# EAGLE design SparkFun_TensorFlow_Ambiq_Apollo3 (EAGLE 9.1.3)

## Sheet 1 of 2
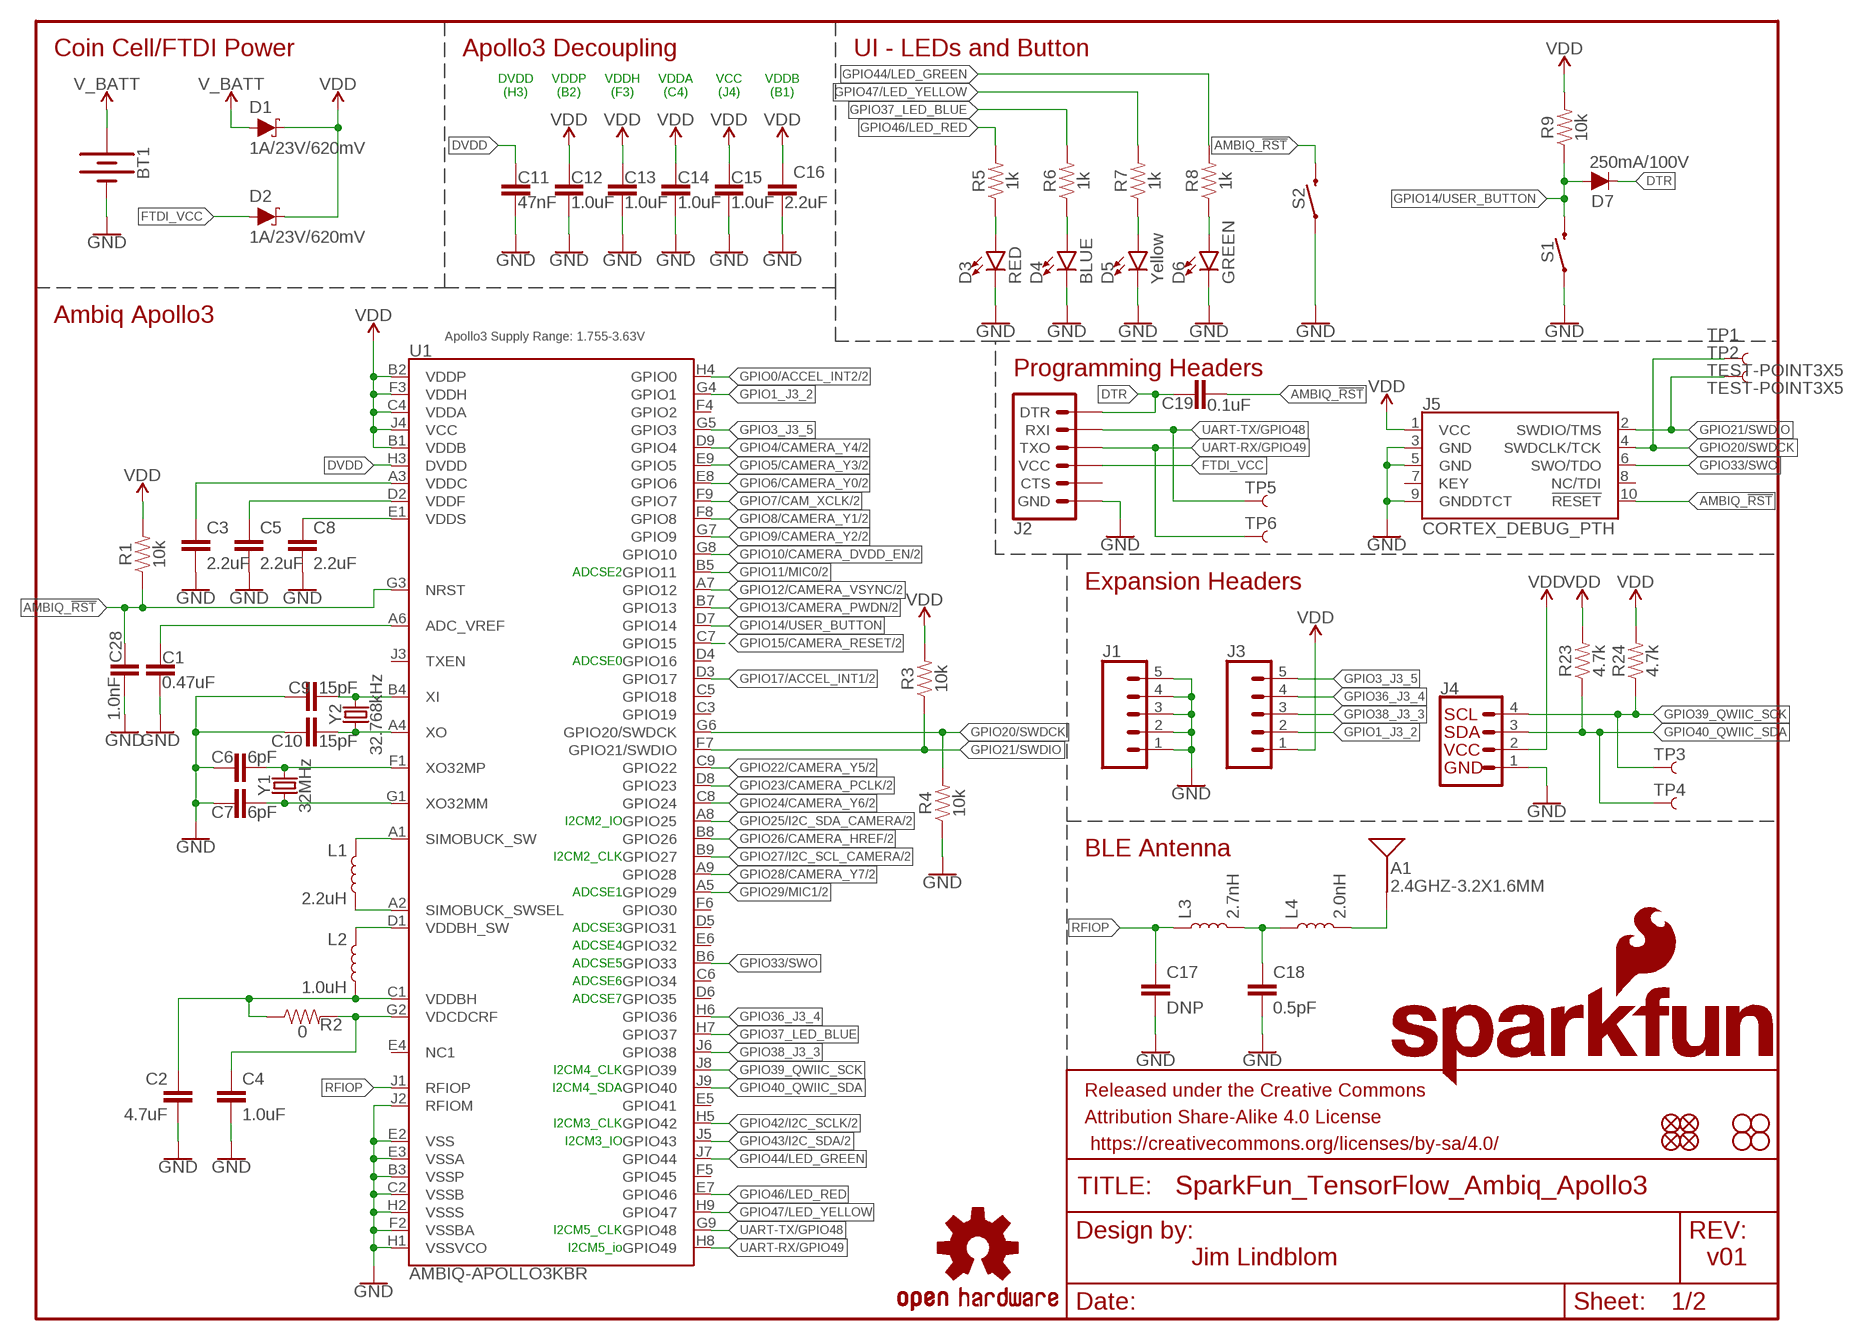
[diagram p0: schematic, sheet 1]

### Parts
A1  2.4GHZ-3.2X1.6MM  ANTENNA-2.4GHZ-3.2X1.6MM  [ANT-2.4GHZ-3.2X1.6X1.2MM]
BT1  BATTERY-20MM_SMD_4LEGS_OVERPASTE_INNER  [BATTCON_20MM_4LEGS_OVERPASTE_INNER]
C1  0.47uF  0.47UF-0402-TIGHT-6.3V-10%  [0402-TIGHT]
C2  4.7uF  4.7UF-0402-TIGHT-6.3V-(20%)  [0402-TIGHT]
C3  2.2uF  2.2UF-0402-TIGHT-25V-10%  [0402-TIGHT]
C4  1.0uF  1.0UF-0402-TIGHT-16V-10%  [0402-TIGHT]
C5  2.2uF  2.2UF-0402-TIGHT-25V-10%  [0402-TIGHT]
C6  6pF  6PF-0402-TIGHT-50V-0.5%  [0402-TIGHT]
C7  6pF  6PF-0402-TIGHT-50V-0.5%  [0402-TIGHT]
C8  2.2uF  2.2UF-0402-TIGHT-25V-10%  [0402-TIGHT]
C9  15pF  15PF-0402-TIGHT-50V-5%  [0402-TIGHT]
C10  15pF  15PF-0402-TIGHT-50V-5%  [0402-TIGHT]
C11  47nF  47NF-0402-TIGHT-25V-10%  [0402-TIGHT]
C12  1.0uF  1.0UF-0402-TIGHT-16V-10%  [0402-TIGHT]
C13  1.0uF  1.0UF-0402-TIGHT-16V-10%  [0402-TIGHT]
C14  1.0uF  1.0UF-0402-TIGHT-16V-10%  [0402-TIGHT]
C15  1.0uF  1.0UF-0402-TIGHT-16V-10%  [0402-TIGHT]
C16  2.2uF  2.2UF-0402-TIGHT-25V-10%  [0402-TIGHT]
C17  DNP  DNP-CAP-0402-TIGHT  [0402-TIGHT]
C18  0.5pF  0.5PF-0402-0.5PF-1%  [0402-TIGHT]
C19  0.1uF  0.1UF-0402-TIGHT-16V-10%  [0402-TIGHT]
C28  1.0nF  1.0NF/1000PF-0402-50V-10%  [0402-TIGHT]
D1  1A/23V/620mV  DIODE-SCHOTTKY-BAT20J  [SOD-323@1]
D2  1A/23V/620mV  DIODE-SCHOTTKY-BAT20J  [SOD-323@1]
D3  RED  LED-RED0603  [LED-0603]
D4  BLUE  LED-BLUE0603  [LED-0603]
D5  Yellow  LED-YELLOW0603  [LED-0603]
D6  GREEN  LED-GREEN0603  [LED-0603]
D7  250mA/100V  DIODE-BAS16J  [SOD-323]
FD1  FIDUCIAL1X2  [FIDUCIAL-1X2]
FD2  FIDUCIAL1X2  [FIDUCIAL-1X2]
FD3  FIDUCIAL1X2  [FIDUCIAL-1X2]
FD4  FIDUCIAL1X2  [FIDUCIAL-1X2]
FRAME1  FRAME-LETTER  [CREATIVE_COMMONS]
H1  STAND-OFF  [STAND-OFF]
H2  STAND-OFF  [STAND-OFF]
H3  STAND-OFF  [STAND-OFF]
H4  STAND-OFF  [STAND-OFF]
J1  CONN_05NO_SILK  [1X05_NO_SILK]
J2  6_PIN_SERIAL_TARGETSMD  [1X06-SMD_RA_MALE]
J3  CONN_05NO_SILK  [1X05_NO_SILK]
J4  QWIIC_CONNECTORJS-1MM  [1X04_1MM_RA]
J5  CORTEX_DEBUG_PTH  [2X5-PTH-1.27MM]
L1  2.2uH  INDUCTOR-0805-2.2UH  [0805-WIDE]
L2  1.0uH  INDUCTOR-0805-1.0UH  [0805-WIDE]
L3  2.7nH  INDUCTOR-0402-2.7NH  [0402-TIGHT]
L4  2.0nH  INDUCTOR-0402-2.0NH  [0402-TIGHT]
LOGO1  SFE_LOGO_NAME_FLAME.1_INCH  [SFE_LOGO_NAME_FLAME_.1]
LOGO2  OSHW-LOGOS  [OSHW-LOGO-S]
R1  10k  10KOHM-0402-TIGHT-1/10W-1%  [0402-TIGHT]
R2  0  0OHM-0402-TIGHT-1/10W-5%  [0402-TIGHT]
R3  10k  10KOHM-0402-TIGHT-1/10W-1%  [0402-TIGHT]
R4  10k  10KOHM-0402-TIGHT-1/10W-1%  [0402-TIGHT]
R5  1k  1KOHM-0603-1/10W-1%  [0603]
R6  1k  1KOHM-0603-1/10W-1%  [0603]
R7  1k  1KOHM-0603-1/10W-1%  [0603]
R8  1k  1KOHM-0603-1/10W-1%  [0603]
R9  10k  10KOHM-0402-TIGHT-1/10W-1%  [0402-TIGHT]
R23  4.7k  4.7KOHM-0603-1/10W-1%  [0603]
R24  4.7k  4.7KOHM-0603-1/10W-1%  [0603]
S1  MOMENTARY-SWITCH-SPST-SMD-5.2-TALL-REDUNDANT  [TACTILE_SWITCH_SMD_5.2MM]
S2  MOMENTARY-SWITCH-SPST-SMD-5.2-TALL-REDUNDANT  [TACTILE_SWITCH_SMD_5.2MM]
TP1  TEST-POINT3X5  [PAD.03X.05]
TP2  TEST-POINT3X5  [PAD.03X.05]
TP3  TEST-POINT3X5  [PAD.03X.05]
TP4  TEST-POINT3X5  [PAD.03X.05]
TP5  TEST-POINT3X5  [PAD.03X.05]
TP6  TEST-POINT3X5  [PAD.03X.05]
U1  AMBIQ-APOLLO3KBR  [BGA-81-5X5MM]
Y1  32MHz  CRYSTAL-32MHZ-SMD-2.0X1.6MM  [CRYSTAL-SMD-2.0X1.6MM]
Y2  32.768kHz  CRYSTAL-32.768KHZSMD-3.2X1.5  [CRYSTAL-SMD-3.2X1.5MM]

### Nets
ADC_VREF: C1.1 U1.A6(ADC_VREF)
AMBIQ_!RST: C19.2 C28.1 J5.10(!RESET) R1.1 S2.3 S2.4 U1.G3(NRST)
DTR: C19.1 D7.C J2.1(DTR)
DVDD: C11.1 U1.H3(DVDD)
FTDI_VCC: D2.A J2.4(VCC)
GND: BT1.2(-) C1.2 C2.2 C3.2 C4.2 C5.2 C6.1 C7.1 C8.2 C9.1 C10.1 C11.2 C12.2 C13.2 C14.2 C15.2 C16.2 C17.2 C18.2 C28.2 D3.C D4.C D5.C D6.C J1.1 J1.2 J1.3 J1.4 J1.5 J2.6(GND) J4.1 J5.3(GND) J5.5(GND) J5.9(GNDDTCT) R4.1 S1.1 S1.2 S2.1 S2.2 U1.B3(VSSP) U1.C2(VSSB) U1.E2(VSS) U1.E3(VSSA) U1.F2(VSSBA) U1.H1(VSSVCO) U1.H2(VSSS) U1.J2(RFIOM) ; also sheet 2
GPIO0/ACCEL_INT2: U1.H4(GPIO0) ; also sheet 2
GPIO1_J3_2: J3.2 U1.G4(GPIO1)
GPIO3_J3_5: J3.5 U1.G5(GPIO3)
GPIO4/CAMERA_Y4: U1.D9(GPIO4) ; also sheet 2
GPIO5/CAMERA_Y3: U1.E9(GPIO5) ; also sheet 2
GPIO6/CAMERA_Y0: U1.E8(GPIO6) ; also sheet 2
GPIO7/CAM_XCLK: U1.F9(GPIO7) ; also sheet 2
GPIO8/CAMERA_Y1: U1.F8(GPIO8) ; also sheet 2
GPIO9/CAMERA_Y2: U1.G7(GPIO9) ; also sheet 2
GPIO10/CAMERA_DVDD_EN: U1.G8(GPIO10) ; also sheet 2
GPIO11/MIC0: U1.B5(GPIO11) ; also sheet 2
GPIO12/CAMERA_VSYNC: U1.A7(GPIO12) ; also sheet 2
GPIO13/CAMERA_PWDN: U1.B7(GPIO13) ; also sheet 2
GPIO14/USER_BUTTON: D7.A R9.1 S1.3 S1.4 U1.D7(GPIO14)
GPIO15/CAMERA_RESET: U1.C7(GPIO15) ; also sheet 2
GPIO17/ACCEL_INT1: U1.D3(GPIO17) ; also sheet 2
GPIO20/SWDCK: J5.4(SWDCLK/TCK) R4.2 TP1.P$1 U1.G6(GPIO20/SWDCK)
GPIO21/SWDIO: J5.2(SWDIO/TMS) R3.1 TP2.P$1 U1.F7(GPIO21/SWDIO)
GPIO22/CAMERA_Y5: U1.C9(GPIO22) ; also sheet 2
GPIO23/CAMERA_PCLK: U1.D8(GPIO23) ; also sheet 2
GPIO24/CAMERA_Y6: U1.C8(GPIO24) ; also sheet 2
GPIO25/I2C_SDA_CAMERA: U1.A8(GPIO25) ; also sheet 2
GPIO26/CAMERA_HREF: U1.B8(GPIO26) ; also sheet 2
GPIO27/I2C_SCL_CAMERA: U1.B9(GPIO27) ; also sheet 2
GPIO28/CAMERA_Y7: U1.A9(GPIO28) ; also sheet 2
GPIO29/MIC1: U1.A5(GPIO29) ; also sheet 2
GPIO33/SWO: J5.6(SWO/TDO) U1.B6(GPIO33)
GPIO36_J3_4: J3.4 U1.H6(GPIO36)
GPIO37_LED_BLUE: R6.2 U1.H7(GPIO37)
GPIO38_J3_3: J3.3 U1.J6(GPIO38)
GPIO39_QWIIC_SCK: J4.4 R24.1 TP3.P$1 U1.J8(GPIO39)
GPIO40_QWIIC_SDA: J4.3 R23.1 TP4.P$1 U1.J9(GPIO40)
GPIO42/I2C_SCLK: U1.H5(GPIO42) ; also sheet 2
GPIO43/I2C_SDA: U1.J5(GPIO43) ; also sheet 2
GPIO44/LED_GREEN: R8.2 U1.J7(GPIO44)
GPIO46/LED_RED: R5.2 U1.E7(GPIO46)
GPIO47/LED_YELLOW: R7.2 U1.H9(GPIO47)
N$1: A1.FEED(SIGNAL) L4.2
N$2: C7.2 U1.G1(XO32MM) Y1.1
N$3: C6.2 U1.F1(XO32MP) Y1.3
N$5: D4.A R6.1
N$6: D3.A R5.1
N$7: D5.A R7.1
N$8: D6.A R8.1
N$16: C18.1 L3.2 L4.1
RFIOP: C17.1 L3.1 U1.J1(RFIOP)
SIMBUCK_SWSEL: L1.2 U1.A2(SIMOBUCK_SWSEL)
SIMOBUCK_SW: L1.1 U1.A1(SIMOBUCK_SW)
UART-RX/GPIO49: J2.3(TXO) TP6.P$1 U1.H8(GPIO49)
UART-TX/GPIO48: J2.2(RXI) TP5.P$1 U1.G9(GPIO48)
V_BATT: BT1.1(+) D1.A
VDCDCRF: C4.1 R2.2 U1.G2(VDCDCRF)
VDD: C12.1 C13.1 C14.1 C15.1 C16.1 D1.C D2.C J3.1 J4.2 J5.1(VCC) R1.2 R3.2 R9.2 R23.2 R24.2 U1.B1(VDDB) U1.B2(VDDP) U1.C4(VDDA) U1.F3(VDDH) U1.J4(VCC) ; also sheet 2
VDDBH: C2.1 L2.2 R2.1 U1.C1(VDDBH)
VDDBH_SW: L2.1 U1.D1(VDDBH_SW)
VDDC: C3.1 U1.A3(VDDC)
VDDF: C5.1 U1.D2(VDDF)
VDDS: C8.1 U1.E1(VDDS)
X0: C10.2 U1.A4(XO) Y2.P$1
XI: C9.2 U1.B4(XI) Y2.P$2
Unconnected: J2.5(CTS) J5.7(KEY) J5.8(NC/TDI) U1.C3(GPIO19) U1.C5(GPIO18) U1.C6(GPIO34) U1.D4(GPIO16) U1.D5(GPIO31) U1.D6(GPIO35) U1.E4(NC1) U1.E5(GPIO41) U1.E6(GPIO32) U1.F4(GPIO2) U1.F5(GPIO45) U1.F6(GPIO30) U1.J3(TXEN)

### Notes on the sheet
- Coin Cell/FTDI Power | Apollo3 Decoupling | UI - LEDs and Button
- DVDD
  (H3)
- VDDP
  (B2)
- VDDH
  (F3)
- VDDA
  (C4)
- VCC
  (J4)
- VDDB
  (B1)
- Ambiq Apollo3
- Apollo3 Supply Range: 1.755-3.63V
- Programming Headers
- ADCSE2 | Expansion Headers
- ADCSE0
- I2CM2_IO
- BLE Antenna
- I2CM2_CLK
- ADCSE1
- ADCSE3
- ADCSE4
- ADCSE5
- ADCSE6
- ADCSE7
- I2CM4_CLK
- I2CM4_SDA
- I2CM3_CLK
- I2CM3_IO
- I2CM5_CLK
- I2CM5_io | Jim Lindblom | v01

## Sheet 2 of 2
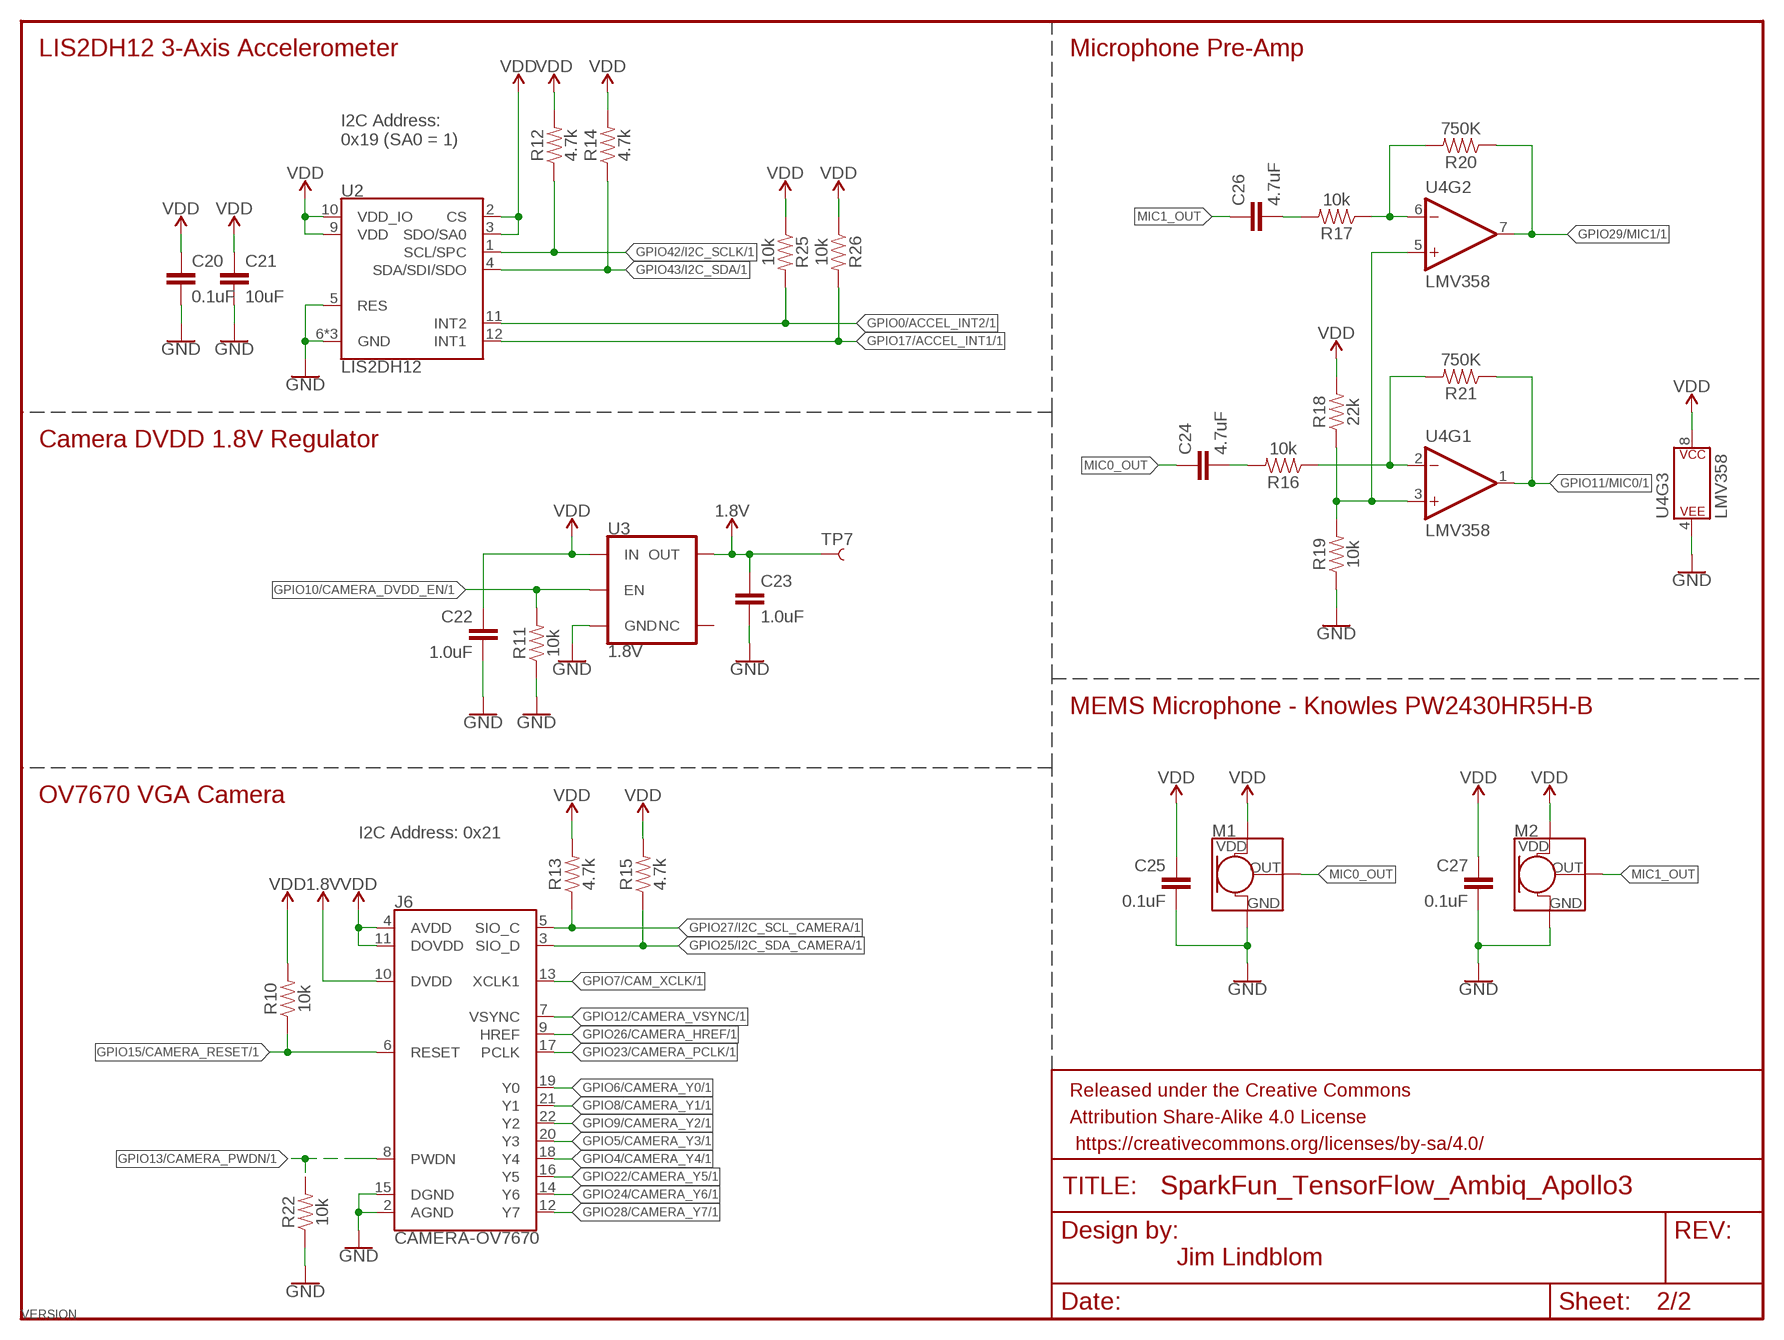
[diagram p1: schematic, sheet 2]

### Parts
C20  0.1uF  0.1UF-0402-TIGHT-16V-10%  [0402-TIGHT]
C21  10uF  10UF-0603-6.3V-20%  [0603]
C22  1.0uF  1.0UF-0402-TIGHT-16V-10%  [0402-TIGHT]
C23  1.0uF  1.0UF-0402-TIGHT-16V-10%  [0402-TIGHT]
C24  4.7uF  4.7UF-0603-6.3V-(10%)  [0603]
C25  0.1uF  0.1UF-0402-TIGHT-16V-10%  [0402-TIGHT]
C26  4.7uF  4.7UF-0603-6.3V-(10%)  [0603]
C27  0.1uF  0.1UF-0402-TIGHT-16V-10%  [0402-TIGHT]
FRAME2  FRAME-LETTERNO_PACKAGE  [DUMMY]
J6  CAMERA-OV7670  [FPC-24-AMPHENOL-SFV24R-1STE1HLF]
M1  MEMS_MIC  MEMS_MICROPHONESPW2430HR5H-B  [SPW2430HR5H-B]
M2  MEMS_MIC  MEMS_MICROPHONESPW2430HR5H-B  [SPW2430HR5H-B]
R10  10k  10KOHM-0402-TIGHT-1/10W-1%  [0402-TIGHT]
R11  10k  10KOHM-0402-TIGHT-1/10W-1%  [0402-TIGHT]
R12  4.7k  4.7KOHM-0603-1/10W-1%  [0603]
R13  4.7k  4.7KOHM-0603-1/10W-1%  [0603]
R14  4.7k  4.7KOHM-0603-1/10W-1%  [0603]
R15  4.7k  4.7KOHM-0603-1/10W-1%  [0603]
R16  10k  10KOHM-0603-1/10W-1%  [0603]
R17  10k  10KOHM-0603-1/10W-1%  [0603]
R18  22k  22KOHM-0402-1/16W-1%  [0402-TIGHT]
R19  10k  10KOHM-0402-TIGHT-1/10W-1%  [0402-TIGHT]
R20  750K  750KOHM-0603-1/10W-1%  [0603]
R21  750K  750KOHM-0603-1/10W-1%  [0603]
R22  10k  10KOHM-0402-TIGHT-1/10W-1%  [0402-TIGHT]
R25  10k  10KOHM-0402-TIGHT-1/10W-1%  [0402-TIGHT]
R26  10k  10KOHM-0402-TIGHT-1/10W-1%  [0402-TIGHT]
TP7  TEST-POINT3X5  [PAD.03X.05]
U2  LIS2DH12  [LGA-12-LISDH12]
U3  1.8V  V_REG_AP2127K-2.8  [SOT23-5]
U4  LMV358  LMV358SOIC  [SO08]

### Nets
1.8V: C23.1 J6.10(DVDD) TP7.P$1 U3.5(OUT)
GND: C20.2 C21.2 C22.2 C23.2 C25.2 C27.2 J6.2(AGND) J6.15(DGND) M1.2(GND) M1.3(GND) M2.2(GND) M2.3(GND) R11.1 R19.1 R22.1 U2.5(RES) U2.6(GND) U2.7(GND) U2.8(GND) U3.2(GND) U4.4(P$V-) ; also sheet 1
GPIO0/ACCEL_INT2: R25.2 U2.11(INT2) ; also sheet 1
GPIO4/CAMERA_Y4: J6.18(Y4) ; also sheet 1
GPIO5/CAMERA_Y3: J6.20(Y3) ; also sheet 1
GPIO6/CAMERA_Y0: J6.19(Y0) ; also sheet 1
GPIO7/CAM_XCLK: J6.13(XCLK1) ; also sheet 1
GPIO8/CAMERA_Y1: J6.21(Y1) ; also sheet 1
GPIO9/CAMERA_Y2: J6.22(Y2) ; also sheet 1
GPIO10/CAMERA_DVDD_EN: R11.2 U3.3(EN) ; also sheet 1
GPIO11/MIC0: R21.1 U4.1(OUT) ; also sheet 1
GPIO12/CAMERA_VSYNC: J6.7(VSYNC) ; also sheet 1
GPIO13/CAMERA_PWDN: J6.8(PWDN) R22.2 ; also sheet 1
GPIO15/CAMERA_RESET: J6.6(RESET) R10.1 ; also sheet 1
GPIO17/ACCEL_INT1: R26.2 U2.12(INT1) ; also sheet 1
GPIO22/CAMERA_Y5: J6.16(Y5) ; also sheet 1
GPIO23/CAMERA_PCLK: J6.17(PCLK) ; also sheet 1
GPIO24/CAMERA_Y6: J6.14(Y6) ; also sheet 1
GPIO25/I2C_SDA_CAMERA: J6.3(SIO_D) R15.1 ; also sheet 1
GPIO26/CAMERA_HREF: J6.9(HREF) ; also sheet 1
GPIO27/I2C_SCL_CAMERA: J6.5(SIO_C) R13.1 ; also sheet 1
GPIO28/CAMERA_Y7: J6.12(Y7) ; also sheet 1
GPIO29/MIC1: R20.1 U4.7(OUT) ; also sheet 1
GPIO42/I2C_SCLK: R12.1 U2.1(SCL/SPC) ; also sheet 1
GPIO43/I2C_SDA: R14.1 U2.4(SDA/SDI/SDO) ; also sheet 1
MIC0_OUT: C24.1 M1.1(OUT)
MIC1_OUT: C26.1 M2.1(OUT)
N$9: R18.1 R19.2 U4.3(+IN) U4.5(+IN)
N$10: C24.2 R16.2
N$11: R17.1 R20.2 U4.6(-IN)
N$12: R16.1 R21.2 U4.2(-IN)
N$14: C26.2 R17.2
VDD: C20.1 C21.1 C22.1 C25.1 C27.1 J6.4(AVDD) J6.11(DOVDD) M1.4(VDD) M2.4(VDD) R10.2 R12.2 R13.2 R14.2 R15.2 R18.2 R25.1 R26.1 U2.2(CS) U2.3(SDO/SA0) U2.9(VDD) U2.10(VDD_IO) U3.1(IN) U4.8(P$V+) ; also sheet 1
Unconnected: J6.MNT1@0(MNT1) J6.MNT1@1(MNT1) J6.MNT2@0(MNT2) J6.MNT2@1(MNT2) U3.4(NC)

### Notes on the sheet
- LIS2DH12 3-Axis Accelerometer | Microphone Pre-Amp
- I2C Address:
  0x19 (SA0 = 1)
- Camera DVDD 1.8V Regulator
- MEMS Microphone - Knowles PW2430HR5H-B
- OV7670 VGA Camera
- I2C Address: 0x21
- Jim Lindblom

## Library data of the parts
A1 = ambiq:ANTENNA: Single-ended Antennae; DIGIKEY: 535-14095-2-ND; PROD_ID: ANT-14235
BT1 = SparkFun-Batteries:BATTERY: Battery - Single Cell
C1 = ambiq:0.47UF: 0.47uF ceramic capacitor; DIGIKEY: 1276-1479-2-ND
C2 = ambiq:4.7UF: 4.7µF ceramic capacitors; DIGIKEY: 1276-1056-1-ND
C3 C5 C8 C16 = ambiq:2.2UF: 2.2µF ceramic capacitors; DIGIKEY: 1276-1462-2-ND
C4 C12-C15 C22 C23 = ambiq:1.0UF: 1µF ceramic capacitors; PROD_ID: CAP-12417
C6 C7 = ambiq:6PF: 6pF ceramic capacitors; PROD_ID: CAP-13455
C9 C10 = ambiq:15PF: 15pF ceramic capacitors; PROD_ID: CAP-13063
C11 = ambiq:47NF: 47nF ceramic capacitors; DIGIKEY: 311-1717-2-ND
C17 = ambiq:DNP-CAP: 0.18µF ceramic capacitor
C18 = ambiq:0.5PF: 0.5pF ceramic capacitor; DIGIKEY: 399-16299-1-ND
C19 C20 C25 C27 = ambiq:0.1UF: 0.1µF ceramic capacitors; PROD_ID: CAP-12416
C21 = SparkFun-Capacitors:10UF: 10.0µF ceramic capacitors; PROD_ID: CAP-11015
C24 C26 = SparkFun-Capacitors:4.7UF: 4.7µF ceramic capacitors; PROD_ID: CAP-08280
C28 = ambiq:1.0NF/1000PF: 1nF/1,000pF ceramic capacitors; DIGIKEY: 311-1036-2-ND
D1 D2 = SparkFun-DiscreteSemi:DIODE-SCHOTTKY: Schottky diode; PROD_ID: DIO-11623
D3 = SparkFun-LED:LED-RED: Red SMD LED; PROD_ID: DIO-00819
D4 = SparkFun-LED:LED-BLUE: Blue SMD LED; PROD_ID: DIO-08575
D5 = SparkFun-LED:LED-YELLOW: Yellow SMD LED; PROD_ID: DIO-09003
D6 = SparkFun-LED:LED-GREEN: Green SMD LED; PROD_ID: DIO-00821
D7 = SparkFun-DiscreteSemi:DIODE: Diode; PROD_ID: DIO-09646
FD1-FD4 = SparkFun-Aesthetics:FIDUCIAL: Fiducial Alignment Points
FRAME1 = SparkFun-Aesthetics:FRAME-LETTER: Schematic Frame - Letter
FRAME2 = SparkFun-Aesthetics:FRAME-LETTER: Schematic Frame - Letter; DESIGNER: Nobody; VERSION: x01
H1-H4 = SparkFun-Hardware:STAND-OFF: Stand Off
J1 J3 = SparkFun-Connectors:CONN_05: Multi connection point. Often used as Generic Header-pin footprint for 0.1 inch spaced/style header connections On any of the 0.1 inch spaced packages, you can populate with these: Break Away Headers - Straight (PRT-00116) Break Away Male Headers - Right Angle (PRT-00553) Female Headers (PRT-00115)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
J2 = SparkFun-Connectors:6_PIN_SERIAL_TARGET: 6-pin header connection for use with the "FTDI BASIC" pinout - TARGET SIDE. Also known as "Arduino Serial Program Header". It is used to mate with our FTDI Basic serial programmers using the Arduino IDE. Note, this device has "TARGET" in the name. It is intended to be used on a design that contains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; PROD_ID: CONN-08971
J4 = SparkFun-Connectors:QWIIC_CONNECTOR: SparkFun I2C Standard Qwiic Connector An SMD 1mm pitch JST connector makes it easy and quick (get it? Qwiic?) to connect I2C devices to each other. The Qwiic system enables fast and solderless connection between popular platforms and various sensors and actuators. We carry 200mm, 100mm, 50mm, and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; PROD_ID: CONN-13694
J5 = SparkFun-Connectors:CORTEX_DEBUG: Cortex Debug Connector - 10 pin Supports JTAG debug, Serial Wire debug, and Serial Wire Viewer. PTH and SMD connector options available. General Connector Information Products: PTH Connector -via Digi-Key SparkFun PSoc SparkFun T
J6 = ambiq:CAMERA-OV7670; DIGIKEY: 609-4320-2-ND
L1 = ambiq:INDUCTOR: Inductors; DIGIKEY: 490-17728-2-ND
L2 = ambiq:INDUCTOR: Inductors; DIGIKEY: 587-2903-2-ND
L3 = ambiq:INDUCTOR: Inductors; DIGIKEY: 445-172420-1-ND
L4 = ambiq:INDUCTOR: Inductors; DIGIKEY: 490-6752-1-ND
LOGO1 = SparkFun-Aesthetics:SFE_LOGO_NAME_FLAME: SparkFun Font Logo w/ Flame
LOGO2 = SparkFun-Aesthetics:OSHW-LOGO: Open-Source Hardware (OSHW) Logo
M1 M2 = ambiq:MEMS_MICROPHONE; DIGIKEY: 423-1394-2-ND
R1 R3 R4 R9-R11 R19 R22 R25 R26 = ambiq:10KOHM: 10kΩ resistor; DIGIKEY: 311-10.0KLRTR-ND
R2 = ambiq:0OHM: 0Ω resistor; DIGIKEY: 311-0.0JRTR-ND
R5-R8 = SparkFun-Resistors:1KOHM: 1kΩ resistor; PROD_ID: RES-07856
R12-R15 R23 R24 = SparkFun-Resistors:4.7KOHM: 4.7kΩ resistor; PROD_ID: RES-07857
R16 R17 = SparkFun-Resistors:10KOHM: 10kΩ resistor; PROD_ID: RES-00824
R18 = ambiq:22KOHM: 22kΩ resistor; DIGIKEY: 311-22.0KLRTR-ND
R20 R21 = SparkFun-Resistors:750KOHM: 750Ω resistor; PROD_ID: RES-13768
S1 S2 = SparkFun-Switches:MOMENTARY-SWITCH-SPST: Momentary Switch (Pushbutton) - SPST; PROD_ID: SWCH-14139
TP1-TP7 = SparkFun-Connectors:TEST-POINT: SparkFun Test Points
U1 = ambiq:AMBIQ-APOLLO3
U2 = ambiq:LIS2DH12; DIGIKEY: 497-14851-2-ND
U3 = ambiq:V_REG_AP2127: Diodes Inc AP2127 -- 300mA LDO Regulator Datasheet; DIGIKEY: AP2127K-1.8TRG1DITR-ND
U4 = SparkFun-IC-Amplifiers:LMV358: IC LMV358 DUAL OP AMP Jellybean rail-to-rail output op-amp SparkFun Products SparkFun PicoBoard (WIG-11888) SparkFun Vernier Interface Shield (DEV-12858) SparkFun Blynk Board - ESP8266 (WRL-13794) SparkFun Digital Sandbox (DEV-12651 RoHS); PROD_ID: IC-09657
Y1 = SparkFun-Clocks:CRYSTAL-32MHZ: 32MHz Crystal; PROD_ID: XTAL-13459
Y2 = SparkFun-Clocks:CRYSTAL-32.768KHZ: 32.768kHz Crystal; PROD_ID: XTAL-13062

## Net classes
0 default: width 0 mm, drill 0 mm
2 usb: width 0.254 mm, drill 0.305 mm, clearance 0.254 mm

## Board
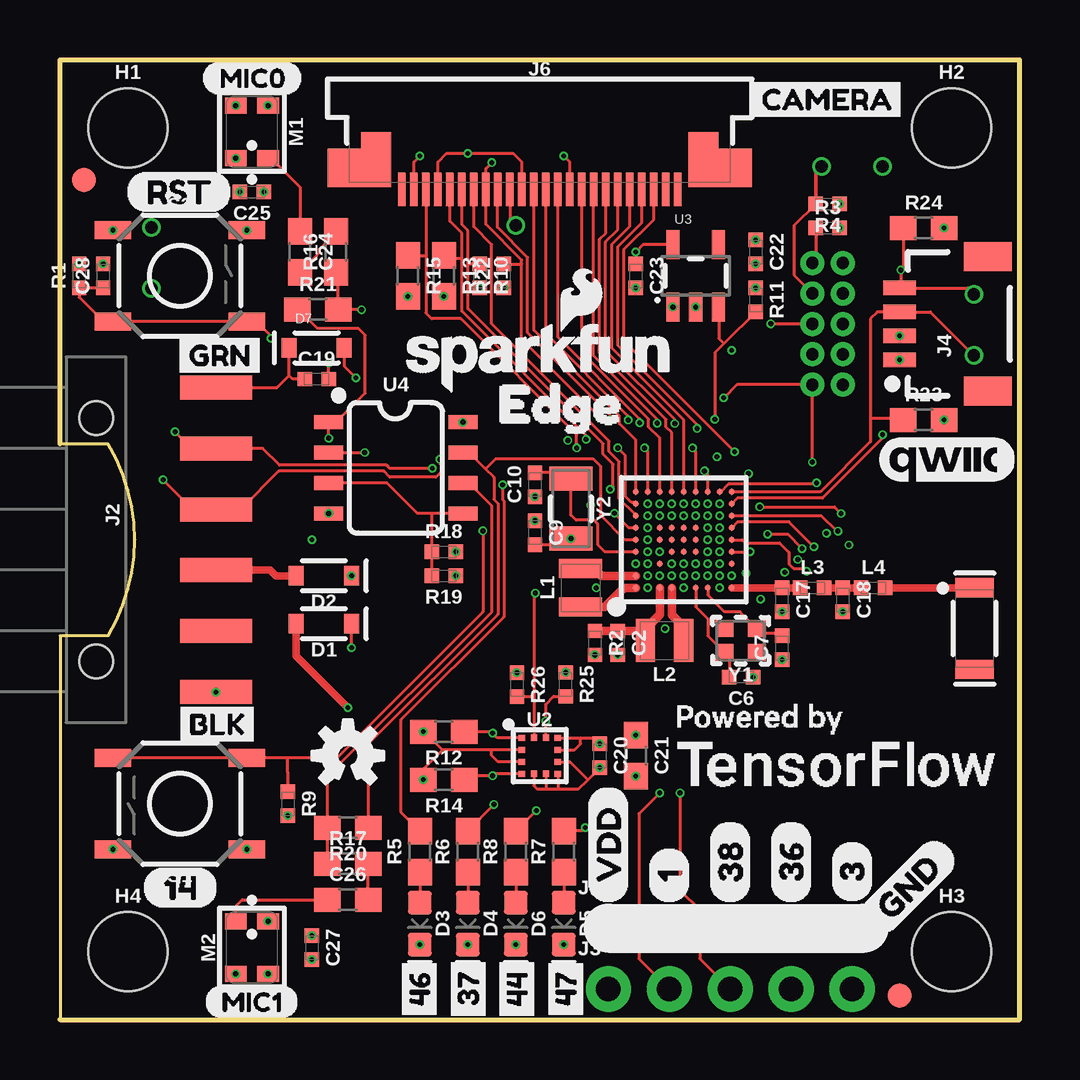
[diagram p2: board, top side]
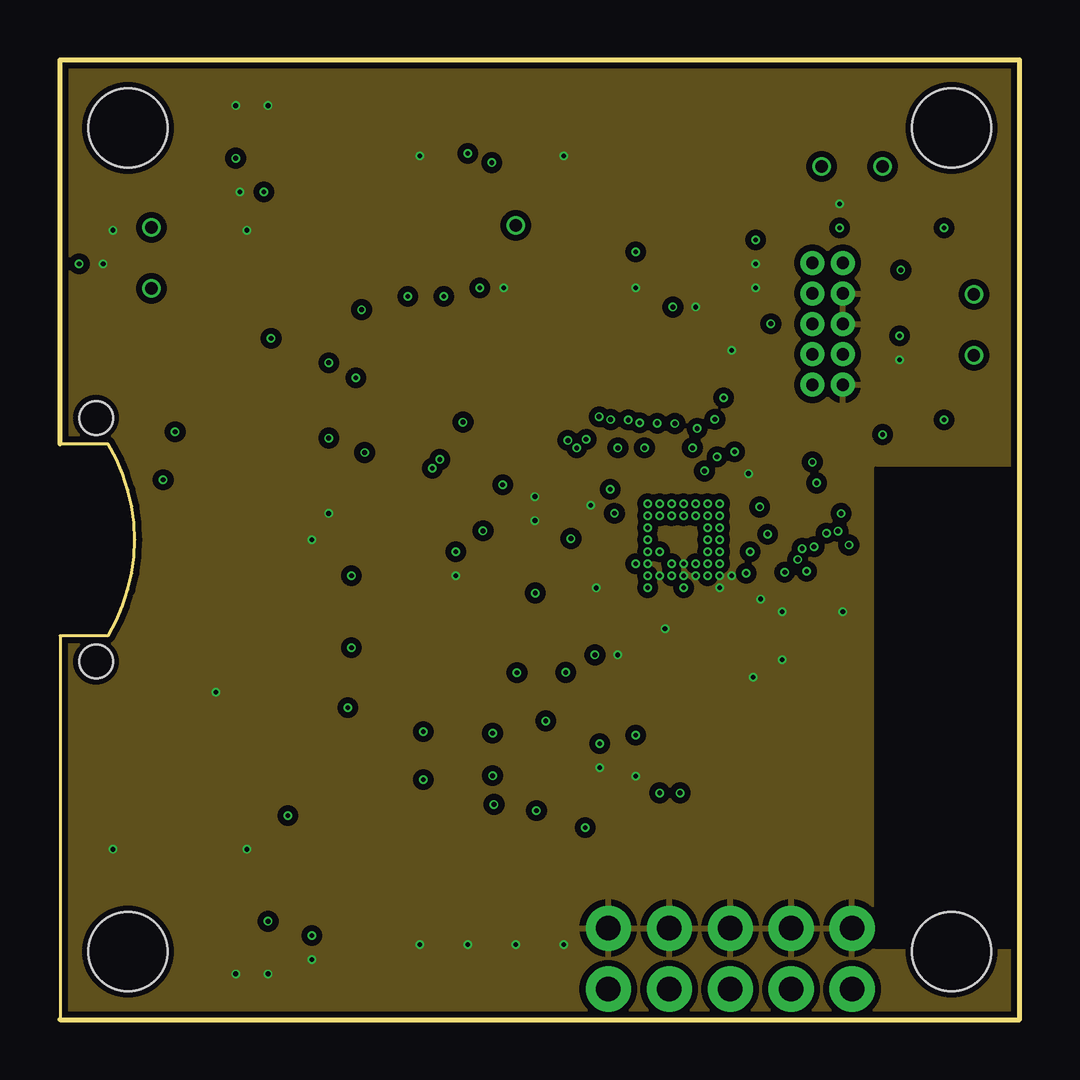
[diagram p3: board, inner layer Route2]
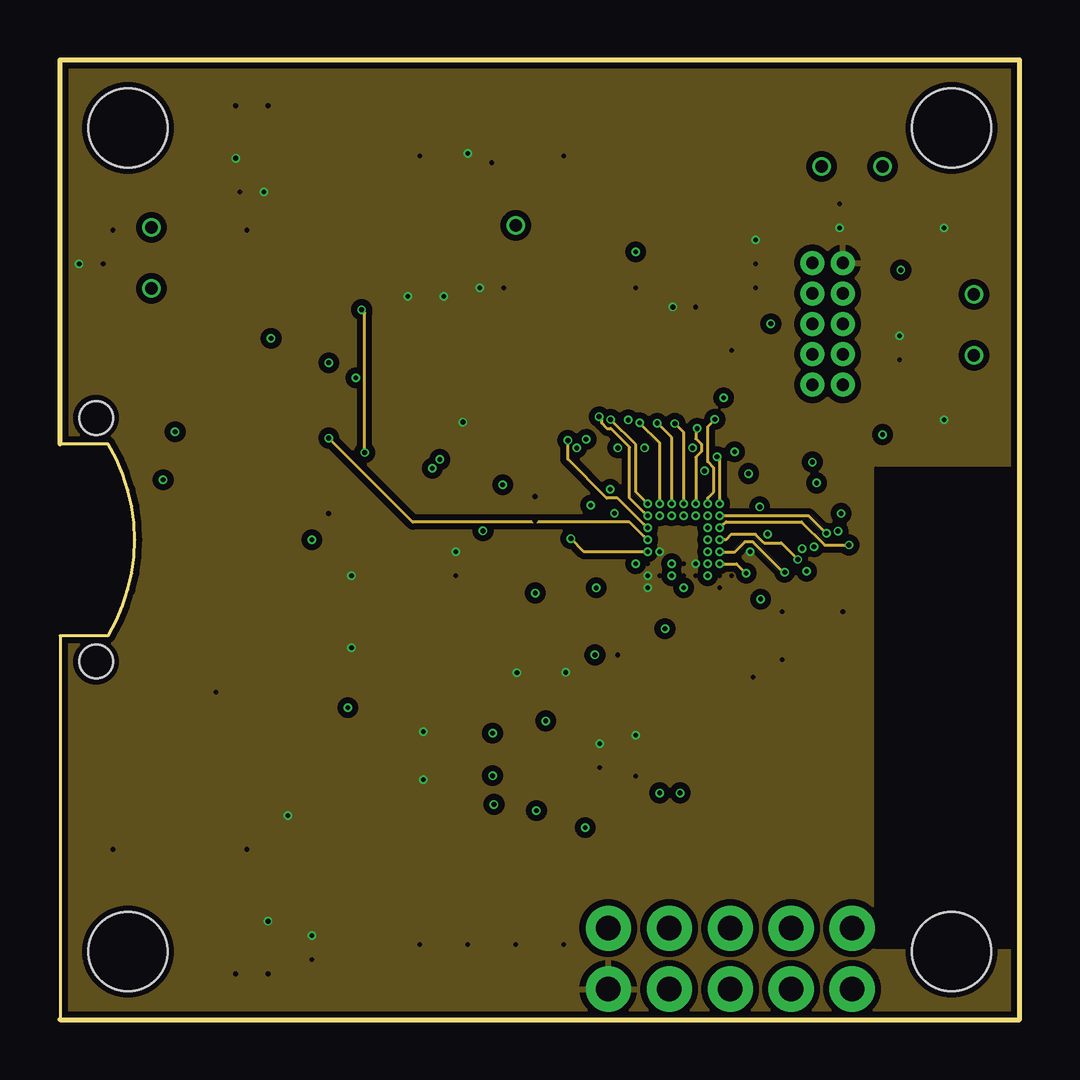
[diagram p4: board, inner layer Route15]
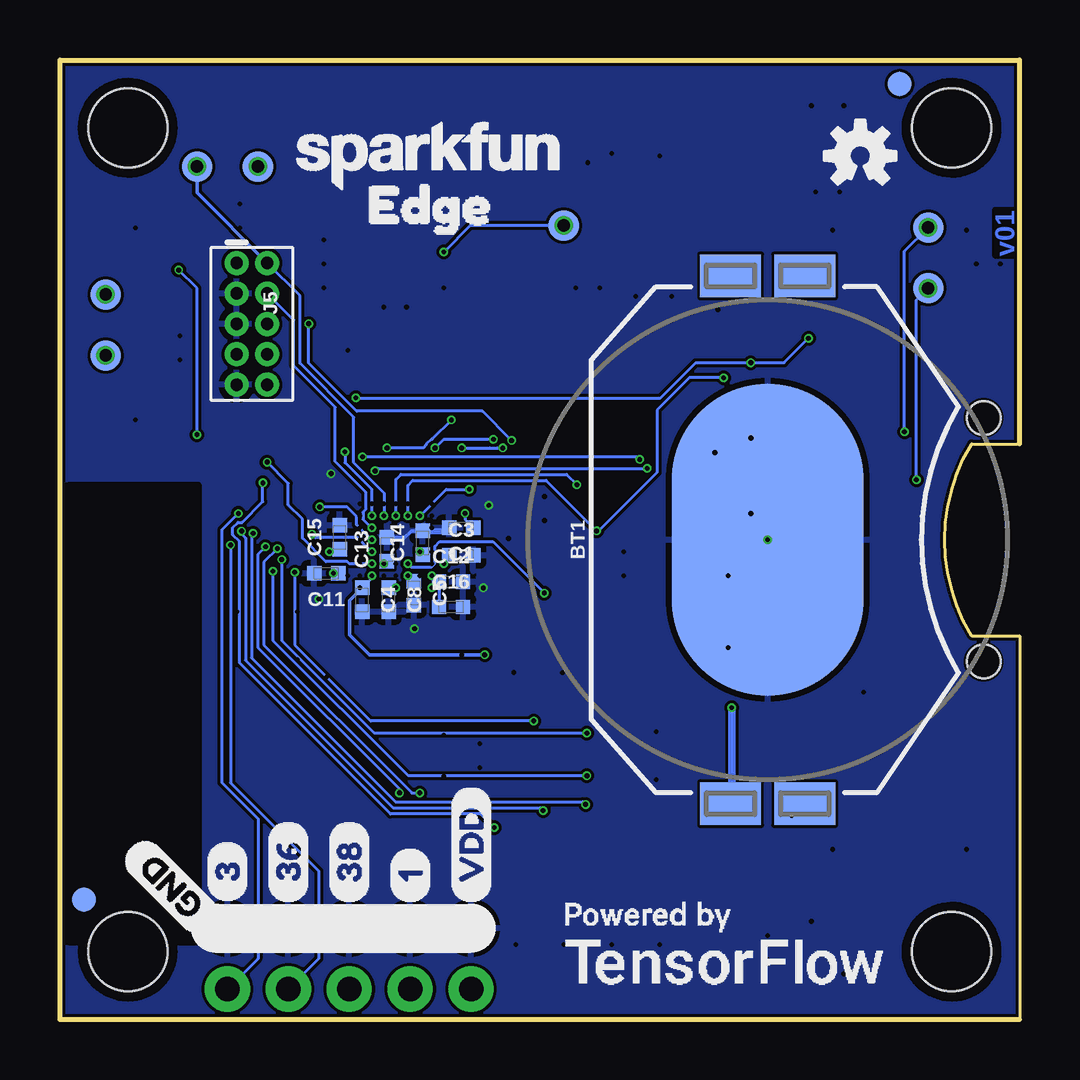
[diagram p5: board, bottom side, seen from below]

Size 40 x 40 mm. Coordinates in mm from the lower left corner, seen from the top.
Outline: 0,0 40,0 40,40 0,40 0,24 2,24 arc-62 2,16 0,16 0,0
Copper layers ([15:(1*2)+15*16]): Top 0.035mm / dielectric 0.213359375mm / Route2 0.035mm / dielectric 1.0161mm / Route15 0.035mm / dielectric 0.213359375mm / Bottom 0.035mm
Design rules "SparkFun-4-layer-PCBWAY-LIMIT": minimum track width 5mil, minimum drill 0.2mm, track to track 5mil, track to pad 5mil, pad to pad 5mil, via to via 5mil, smd to smd 0mil, copper to edge 5mil, drill to drill 5mil, minimum pad ring 3mil, minimum via ring 3mil, stop-mask expansion 4mil, vias tented up to drill 25mil, thermal gap 10mil

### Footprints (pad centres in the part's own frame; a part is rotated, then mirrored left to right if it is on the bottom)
ANT-2.4GHZ-3.2X1.6X1.2MM = smd 0.8 x 1.6: FEED -1.7,0; NC 1.7,0
BATTCON_20MM_4LEGS_OVERPASTE_INNER = smd 1.778 x 2.54: 1 -11,1.55; 3 11,1.55; P$1 -11,-1.55; P$2 11,-1.55 | smd 13 x 8: 2 0,0
0402-TIGHT = smd 0.6 x 0.6: 1 -0.5,0; 2 0.5,0
0603 = smd 1.1 x 1: 1 -0.85,0; 2 0.85,0
SOD-323@1 = smd 0.63 x 0.83: A 1.15,0; C -1.15,0
LED-0603 = smd 1 x 1: A -0.877,0; C 0.877,0
SOD-323 = smd 0.63 x 0.83: A 1.15,0; C -1.15,0
FIDUCIAL-1X2 = smd 1 x 1: 1 0,0
STAND-OFF = hole 3.302: 0,0
1X05_NO_SILK = drill 1.016 pad 1.88: 1 0,0; 2 2.54,0; 3 5.08,0; 4 7.62,0; 5 10.16,0
1X06-SMD_RA_MALE = smd 1 x 3: 1 -6.35,5; 2 -3.81,5; 3 -1.27,5; 4 1.27,5; 5 3.81,5; 6 6.35,5 | hole 1.4: -5.08,0; 5.08,0
1X04_1MM_RA = smd 0.6 x 1.35: 1 -1.5,0; 2 -0.5,0; 3 0.5,0; 4 1.5,0 | smd 1.2 x 2: NC1 2.8,-3.675; NC2 -2.8,-3.675
2X5-PTH-1.27MM = drill 0.508 pad 1: 1 -2.54,-0.635; 2 -2.54,0.635; 3 -1.27,-0.635; 4 -1.27,0.635; 5 0,-0.635; 6 0,0.635; 7 1.27,-0.635; 8 1.27,0.635; 9 2.54,-0.635; 10 2.54,0.635
FPC-24-AMPHENOL-SFV24R-1STE1HLF = smd 0.3 x 1.4: 1 5.75,2.4; 2 5.25,2.4; 3 4.75,2.4; 4 4.25,2.4; 5 3.75,2.4; 6 3.25,2.4; 7 2.75,2.4; 8 2.25,2.4; 9 1.75,2.4; 10 1.25,2.4; 11 0.75,2.4; 12 0.25,2.4; 13 -0.25,2.4; 14 -0.75,2.4; 15 -1.25,2.4; 16 -1.75,2.4; 17 -2.25,2.4; 18 -2.75,2.4; 19 -3.25,2.4; 20 -3.75,2.4; 21 -4.25,2.4; 22 -4.75,2.4; 23 -5.25,2.4; 24 -5.75,2.4 | smd 1.4 x 1.6: MNT1@0 -8.15,1.5; MNT2@1 8.15,1.5 | smd 1.25 x 2.3: MNT1@1 -6.825,1.15; MNT2@0 6.825,1.15
0805-WIDE = smd 0.8 x 1.8: 1 -0.8,0; 2 0.8,0
SPW2430HR5H-B = smd 0.9 x 0.66: 1 -0.675,1.095; 2 -0.675,-1.095; 3 0.675,-1.095; 4 0.675,1.095
TACTILE_SWITCH_SMD_5.2MM = smd 1.524 x 0.762: 1 -2.794,1.905; 2 2.794,1.905; 3 -2.794,-1.905; 4 2.794,-1.905
PAD.03X.05 = smd 1.27 x 1.27: P$1 0,0
BGA-81-5X5MM = smd 0.254 x 0.254: A1 -2,2; A2 -1.5,2; A3 -1,2; A4 -0.5,2; A5 0,2; A6 0.5,2; A7 1,2; A8 1.5,2; A9 2,2; B1 -2,1.5; B2 -1.5,1.5; B3 -1,1.5; B4 -0.5,1.5; B5 0,1.5; B6 0.5,1.5; B7 1,1.5; B8 1.5,1.5; B9 2,1.5; C1 -2,1; C2 -1.5,1; C3 -1,1; C4 -0.5,1; C5 0,1; C6 0.5,1; C7 1,1; C8 1.5,1; C9 2,1; D1 -2,0.5; D2 -1.5,0.5; D3 -1,0.5; D4 -0.5,0.5; D5 0,0.5; D6 0.5,0.5; D7 1,0.5; D8 1.5,0.5; D9 2,0.5; E1 -2,0; E2 -1.5,0; E3 -1,0; E4 -0.5,0; E5 0,0; E6 0.5,0; E7 1,0; E8 1.5,0; E9 2,0; F1 -2,-0.5; F2 -1.5,-0.5; F3 -1,-0.5; F4 -0.5,-0.5; F5 0,-0.5; F6 0.5,-0.5; F7 1,-0.5; F8 1.5,-0.5; F9 2,-0.5; G1 -2,-1; G2 -1.5,-1; G3 -1,-1; G4 -0.5,-1; G5 0,-1; G6 0.5,-1; G7 1,-1; G8 1.5,-1; G9 2,-1; H1 -2,-1.5; H2 -1.5,-1.5; H3 -1,-1.5; H4 -0.5,-1.5; H5 0,-1.5; H6 0.5,-1.5; H7 1,-1.5; H8 1.5,-1.5; H9 2,-1.5; J1 -2,-2; J2 -1.5,-2; J3 -1,-2; J4 -0.5,-2; J5 0,-2; J6 0.5,-2; J7 1,-2; J8 1.5,-2; J9 2,-2
LGA-12-LISDH12 = smd 0.275 x 0.25: 1 -0.75,0.75; 2 -0.75,0.25; 3 -0.75,-0.25; 4 -0.75,-0.75; 7 0.75,-0.75; 8 0.75,-0.25; 9 0.75,0.25; 10 0.75,0.75 | smd 0.25 x 0.275: 5 -0.25,-0.75; 6 0.25,-0.75; 11 0.25,0.75; 12 -0.25,0.75
SOT23-5 = smd 0.55 x 1.2: 1 -0.95,-1.3; 2 0,-1.3; 3 0.95,-1.3; 4 0.95,1.3; 5 -0.95,1.3
SO08 = smd 0.6 x 1.2: 1 -1.905,-2.8; 2 -0.635,-2.8; 3 0.635,-2.8; 4 1.905,-2.8; 5 1.905,2.8; 6 0.635,2.8; 7 -0.635,2.8; 8 -1.905,2.8
CRYSTAL-SMD-2.0X1.6MM = smd 0.75 x 0.7: 1 -0.675,-0.5; 2 0.675,-0.5; 3 0.675,0.5; 4 -0.675,0.5
CRYSTAL-SMD-3.2X1.5MM = smd 1 x 1.8: P$1 -1.25,0; P$2 1.25,0

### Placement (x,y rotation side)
A1  38.13,16.3 270 top
BT1  10.5,20 90 bottom
C1  23.27,20.5 180 bottom
C2  23.25,15.7 270 top
C3  23.27,19.35 0 bottom
C4  27.4,17.5 270 bottom
C5  25.25,17.77 270 bottom
C6  28.4,14.27 180 top
C7  30.1,15.5 90 top
C8  26.3,17.5 270 bottom
C9  19.8,20.3 270 top
C10  19.8,22.3 90 top
C11  28.9,18.6 180 bottom
C12  23.7,18.25 0 bottom
C13  26.37,19.6 90 bottom
C14  24.88,19.87 90 bottom
C15  28.34,20.1 90 bottom
C16  23.7,17.2 0 bottom
C17  30.1,17.5 270 top
C18  32.63,17.5 270 top
C19  10.7,26.7 0 top
C20  22.5,11 270 top
C21  24,11 270 top
C22  29,32 270 top
C23  24,31 270 top
C24  10,32 270 top
C25  8,34.5 180 top
C26  12,5 0 top
C27  10.5,3 270 top
C28  1.8,31 90 top
D1  11,16.5 180 top
D2  11,18.5 180 top
D3  15,4 270 top
D4  17,4 270 top
D5  21,4 270 top
D6  19,4 270 top
D7  10.7,28 0 top
FD1  1,35 0 top
FD2  35,1 0 top
FD3  39,5 0 bottom
FD4  5,39 0 bottom
FRAME1  not placed on the board
FRAME2  not placed on the board
H1  2.83,37.17 0 top
H2  37.17,37.17 0 top
H3  37.17,2.83 0 top
H4  2.83,2.83 0 top
J1  22.86,3.81 0 top
J2  1.5,20 270 top
J3  22.86,1.27 0 top
J4  35,29 90 top
J5  32,29 270 bottom
J6  20,37 180 top
L1  21.7,18 90 top
L2  25.2,15.8 180 top
L3  31.36,18 0 top
L4  33.9,18 0 top
LOGO1  20,27.6 0 top
LOGO2  12,11 0 top
M1  8,37 180 top
M2  8,3 0 top
R1  0.8,31 90 top
R2  22.3,15.7 270 top
R3  32,33 0 top
R4  32,34 180 top
R5  15,7 90 top
R6  17,7 90 top
R7  21,7 90 top
R8  19,7 90 top
R9  9.5,9 270 top
R10  17.5,31 270 top
R11  29,30 270 top
R12  16,12 180 top
R13  16,31 270 top
R14  16,10 180 top
R15  14.5,31 270 top
R16  11.5,32 90 top
R17  12,6.5 0 top
R18  16,19.5 0 top
R19  16,18.5 180 top
R20  12,8 180 top
R21  10.75,29.6 0 top
R22  18.5,31 90 top
R23  36,25 0 top
R24  36,33 0 top
R25  21.08,13.97 270 top
R26  19.05,13.96 270 top
S1  5,9 180 top
S2  5,31 0 top
TP1  31.75,35.56 0 bottom
TP2  34.29,35.56 0 bottom
TP3  38.1,30.23 0 bottom
TP4  38.1,27.69 0 bottom
TP5  3.81,33.02 0 bottom
TP6  3.81,30.48 0 bottom
TP7  19,33.1 0 bottom
U1  26,20 90 top
U2  20,11 0 top
U3  26.5,31 0 top
U4  14,23 270 top
U$1  [MIC00]  5.92,39.24 0 top
U$2  [BLK2]  4.57,12.32 0 top
U$3  [GND0]  33.66,3.81 45 top
U$4  [VDD1]  22.86,4.83 90 top
U$5  [10]  25.4,4.83 90 top
U$6  [383]  27.94,4.83 90 top
U$7  [364]  30.48,4.83 90 top
U$8  [10]  25.4,4.83 90 bottom
U$9  [VDD1]  22.86,4.83 90 bottom
U$10  [31]  33.02,4.83 90 bottom
U$11  [383]  27.94,4.83 90 bottom
U$12  [364]  30.48,4.83 90 bottom
U$13  [31]  33.02,4.83 90 top
U$14  [GND0]  33.66,3.81 135 bottom
U$15  [461]  14.99,-0.25 90 top
U$16  [372]  17.02,-0.25 90 top
U$17  [443]  19.05,-0.25 90 top
U$18  [470]  21.08,-0.25 90 top
U$19  [QWIIC_COPYRIGHT_SMALL]  36.96,23.37 0 top
U$20  [CAMERA3]  28.45,38.35 0 top
U$21  [POWEREDBY_TF#JPG]  32.26,11.68 0 top
U$22  [MIC11]  5.99,0.74 0 top
U$23  [EDGE0]  28.56,33.96 0 bottom
U$24  [EDGE0]  16.89,25.65 0 top
U$25  [POWEREDBY_TF#JPG]  12.4,3.45 0 bottom
U$26  [1416]  3.4,5.5 0 top
U$27  [RST15]  2.7,34.5 0 top
U$28  [GRN1]  4.57,27.69 0 top
U$29  [SFE_LOGO_NAME_.1]  24.64,36 0 bottom
U$30  [OSHW-LOGO-S]  6.64,36 0 bottom
Y1  28.37,15.8 180 top
Y2  21.3,21.3 270 top

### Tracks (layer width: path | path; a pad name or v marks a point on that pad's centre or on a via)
1.8V  (via drill 0.2 pad 0.25, 0.51 pad 0.25)
  Top 0.127: J6.10 18.75,33.35 TP7.P$1 | C23.1 v24,32 24.3,32.3 U3.5
  Bottom 0.127: TP7.P$1 22.9,33.1 v24,32
  other vias: 19,33.1
ADC_VREF  (via drill 0.2)
  Top 0.127: U1.A6 23.72,20.5 v23.11,21.1
  Bottom 0.127: v23.11,21.1 23.11,20.84 C1.1
AMBIQ_!RST  (via drill 0.2)
  Top 0.127: v27.67,25.91 28.21,26.46 J5.10 v31.36,23.24 | C28.1 R1.1 0.8,30.11 1.82,29.09 S2.3 S2.4 8.21,29.09 8.8,28.5 v8.8,28.4 | C19.2 v11.2,27.38
  Bottom 0.127: v31.36,23.24 30.48,22.35 30.48,21.45 29.9,20.86 29.9,20.07 28.92,19.09 28.02,19.09 27.93,19 U1.G3 | v27.67,25.91 14.96,25.91 13.49,27.38 v11.2,27.38 9.82,27.38 v8.8,28.4
  other vias: 27,19
CUTOUT
  cutout Route15 (isolate 0.152): 34,23 40,23 40,3 34,3
  cutout Route2 (isolate 0.152): 34,23 40,23 40,3 34,3
DTR
  Top 0.127: J2.1 9.05,26.35 9.55,26.85 | 9.55,26.85 D7.C | C19.1 9.7,26.7 9.55,26.85
DVDD  (via drill 0.2, 0.2 layers 1-15)
  Route15 0.127: U1.H3 28.2,19 v28.6,18.6
  Bottom 0.127: v28.6,18.6 C11.1
  other vias: 27.5,19
FTDI_VCC
  Top 0.127: 9.9,18.5 D2.A
  Top 0.305: J2.4 8.77,18.73 9,18.5 D2.A
GND  (via drill 0.2, 0.2 layers 1-2, 0.2 pad 0.25, 0.2 pad 0.25 layers 1-2)
  Top 0.127: U2.5 19.75,9.75 19.9,9.6 20.3,9.6 | 20.8,9.6 21.6,9.6 22,10 | 20.8,9.6 20.3,9.6 | 22,10 C20.2 | U2.6 20.25,9.65 20.3,9.6 | U2.7 20.75,9.65 20.8,9.6 | U2.8 21.25,10.75 22,10 | J6.15 21.25,35.75 v21,36 | J6.2 14.75,35.75 v15,36
  Bottom 0.127: BT1.2 10.5,20.28
  Bottom 0.152: C13.2 25.69,20.1 25.65,20.07 25.35,20.37 C14.2
  Bottom 0.254: C14.2 23.9,20.37 C1.2
  other vias: 27.5,18 27.5,18.5 28,18.5 26.5,18.5 26,18.5 26,19 25,18.5 24.5,19 28.9,14.27 30.1,15 32.63,17 30.1,17 19.8,21.8 19.8,20.8 7.33,38.09 8.68,38.09 7.5,34.5 7.79,32.91 2.21,32.91 16.5,18.5 11.2,21.09 10.5,20 6.5,13.65 7.79,7.09 2.21,7.09 7.33,1.91 8.68,1.91 10.5,2.5 15,3.12 17,3.12 29,31.5 26.5,29.7 24,30.5 22.5,10.5 24,10.15 28,27.9 29,30.5 18.5,30.5 35,27.5 32.5,34 21,3.12 19,3.12 28.7,22.76 29.21,17.53 22.35,17.99 25.22,16.29 22.12,21.44 23.25,15.2 1.8,31.5
  pour Route2 (isolate 0.254, rank 6): 0,40 0,0 40,0 40,40
  pour Bottom (isolate 0.127): 0,40 0,0 40,0 40,40
GPIO0/ACCEL_INT2  (via drill 0.2, 0.2 layers 1-15)
  Top 0.127: U2.11 v20.25,12.45 20.25,13.14 20.58,13.47 R25.2
  Route15 0.127: U1.H4 28.14,19.5 28.55,19.92 28.89,19.92 30.16,18.64 v30.21,18.64
  Bottom 0.127: 30.21,18.43 v30.21,18.64 30.21,15.62 27.05,12.45 v20.25,12.45
  other vias: 27.5,19.5
GPIO1_J3_2  (via drill 0.2)
  Top 0.127: v29.5,20.23 30.34,20.23 v30.94,19.63 | v25,9.45 24.13,8.58 24.13,2.54 J3.2
  Bottom 0.127: U1.G4 27.13,19.63 27.15,19.63 27.37,19.85 27.37,19.87 27.59,20.09 29.36,20.09 v29.5,20.23 | v30.94,19.63 31.5,19.07 31.5,15.62 25.33,9.45 v25,9.45
  other vias: 27,19.5
GPIO3_J3_5  (via drill 0.2)
  Top 0.127: v32.56,21.09 32.29,21.37 v29.17,21.37
  Bottom 0.127: U1.G5 27.13,20.13 27.15,20.13 27.64,20.63 27.64,20.98 28.03,21.37 v29.17,21.37 | J3.5 31.75,2.54 31.75,8.38 33.25,9.88 33.25,20.41 32.69,20.98 32.67,20.98 v32.56,21.09
  other vias: 27,20
GPIO4/CAMERA_Y4
  Top 0.127: 22.67,34.52 J6.18 22.75,32.79 22.49,32.53 22.49,27.79 25.27,25.01 25.27,24.69 25.5,24.46 U1.D9
GPIO5/CAMERA_Y3
  Top 0.127: U1.E9 26,25 23,28 23,32.32 23.75,33.07 J6.20
GPIO6/CAMERA_Y0  (via drill 0.2 layers 1-15)
  Top 0.127: v25.63,24.84 25.63,25 22.75,27.89 22.75,32.42 23.25,32.93 J6.19
  Route15 0.127: v25.63,24.84 26,24.48 U1.E8
  other vias: 26,21.5
GPIO7/CAM_XCLK  (via drill 0.2)
  Top 0.127: U1.F9 26.5,23.7 v26.37,23.83 | v23.69,25 23.69,25.15 20.25,28.59 J6.13
  Bottom 0.127: v26.37,23.83 24.85,23.83 24.73,23.95 24.73,23.98 24.52,24.2 24.49,24.2 v23.69,25
GPIO8/CAMERA_Y1  (via drill 0.2 layers 1-15)
  Top 0.127: J6.21 24.26,33.22 23.26,32.22 23.26,28.1 26.56,24.8 v26.56,24.64
  Route15 0.127: v26.56,24.64 26.5,24.58 26.5,24.21 26.73,23.98 26.73,23.68 26.5,23.44 U1.F8
  other vias: 26.5,21.5
GPIO9/CAMERA_Y2  (via drill 0.2)
  Top 0.127: v28.12,23.67 23.51,28.28 23.51,32.11 24.75,33.35 J6.22
  Bottom 0.127: U1.G7 27,22.09 28.12,23.22 v28.12,23.67
  other vias: 27,21
GPIO10/CAMERA_DVDD_EN  (via drill 0.2 layers 1-15)
  Top 0.127: U3.3 27.46,28.39 27.65,28.2 27.7,28.2 | R11.2 27.7,28.2 | 27.7,28.2 27.3,27.8 v27.3,25.02
  Route15 0.127: U1.G8 27,21.74 27.25,22 27.25,23 27,23.25 27,24.72 v27.3,25.02
  other vias: 27,21.5
GPIO11/MIC0  (via drill 0.2 layers 1-15)
  Top 0.127: v11.2,24.24 U4.1 11.52,24.91 12.72,26.11 12.72,28.52 12.45,28.8 10.74,28.8 9.95,29.6 R21.1
  Route15 0.127: v11.2,24.24 14.7,20.74 23.75,20.74 24.35,20.13 24.37,20.13 U1.B5
  other vias: 24.5,20
GPIO12/CAMERA_VSYNC
  Top 0.127: J6.7 17.25,33.05 17.99,32.31 17.99,29.01 22.89,24.11 22.89,23.68 23.31,23.26 23.31,21.71 24,21.02 U1.A7
GPIO13/CAMERA_PWDN  (via drill 0.2 layers 1-15, 0.2 pad 0.25 layers 1-2)
  Top 0.127: v18,35.72 17.75,35.47 J6.8 17.75,33.15 19.24,31.66 19.24,31.5 | R22.2 19.24,31.5 | v22.47,25.13 19.24,28.36 19.24,31.5
  Route15 0.127: v22.47,25.13 22.59,25.02 22.59,24.86 22.8,24.64 22.96,24.64 23.75,23.86 23.75,21.73 24.35,21.13 24.37,21.13 U1.B7
  other vias: 24.5,21
GPIO14/USER_BUTTON  (via drill 0.2)
  Top 0.127: R9.1 9.5,10.31 | S1.4 S1.3 9.5,10.9 | 9.5,10.9 11.55,10.9 17.63,16.99 v17.63,20.37 | 9.5,10.31 | 9.5,10.31 9.5,10.9 | D7.A 11.85,27.24 v12.33,26.75
  Bottom 0.127: U1.D7 25.5,22.27 25.3,22.47 19.73,22.47 v17.63,20.37 17.55,20.37 15.11,22.81 15.11,25.4 13.76,26.75 v12.33,26.75
  other vias: 25.5,21
GPIO15/CAMERA_RESET  (via drill 0.2)
  Top 0.127: v22.94,22.1 23.05,22.22 23.05,23.15 22.64,23.57 22.64,24 17.01,29.63 17.01,31.5 | J6.6 16.75,33.14 17.01,32.88 17.01,31.5 | R10.1 17.01,31.5
  Bottom 0.127: U1.C7 23.9,22.1 v22.94,22.1
  other vias: 25,21
GPIO17/ACCEL_INT1  (via drill 0.2)
  Top 0.127: v19.81,17.78 19.75,17.72 19.75,13.46 | 19.75,13.46 U2.12 | R26.2 19.75,13.46
  Bottom 0.127: U1.D3 25.37,18.87 24.51,18.87 24.37,19.02 24.37,19.73 24.17,19.92 21.95,19.92 v19.81,17.78
  other vias: 25.5,19
GPIO20/SWDCK  (via drill 0.2 pad 0.25, 0.51)
  Top 0.127: R4.2 30.6,33.1 30.6,31.04 J5.4
  Top 0.152: R4.2 31.5,35.31 TP1.P$1
  Bottom 0.127: U1.G6 27.13,20.63 27.15,20.63 27.37,20.85 27.37,21.15 27.25,21.27 27.25,21.99 28.52,23.26 28.52,25.52 30.25,27.25 30.25,29.16 J5.4
  other vias: 27,20.5 31.75,35.56
GPIO21/SWDIO  (via drill 0.2 pad 0.25, 0.51)
  Top 0.127: R3.1 31.5,31.68 J5.2
  Bottom 0.127: U1.F7 26.5,21.95 27.76,23.21 27.76,25.11 30,27.36 30,30.18 J5.2
  Bottom 0.152: J5.2 34.29,34.47 TP2.P$1
  other vias: 26.5,21 34.29,35.56
GPIO22/CAMERA_Y5
  Top 0.127: U1.C9 25,24.24 24.53,24.71 24.53,25.03 21.75,27.81 J6.16
GPIO23/CAMERA_PCLK  (via drill 0.2 layers 1-15)
  Top 0.127: J6.17 | v24.9,24.86 24.9,25.02 22.24,27.68 22.24,34.59 J6.17
  Route15 0.127: U1.D8 25.5,24.26 v24.9,24.86
  other vias: 25.5,21.5
GPIO24/CAMERA_Y6  (via drill 0.2 layers 1-15)
  Top 0.127: J6.14 20.75,28.45 24.17,25.03 v24.17,24.88
  Route15 0.127: U1.C8 25,24.04 v24.17,24.88
  other vias: 25,21.5
GPIO25/I2C_SDA_CAMERA  (via drill 0.2)
  Top 0.127: U1.A8 24,21.54 23.98,21.56 23.82,21.56 23.56,21.82 23.56,23.52 v23.26,23.83 | J6.3 15.25,31.85 | 15.25,31.85 15.25,29.45 15.49,29.21 16.71,29.21 21.54,24.38 v21.54,23.83 | R15.1 15.25,31.85
  Bottom 0.127: v23.26,23.83 22.09,23.83 22.08,23.82 21.78,23.82 21.77,23.83 v21.54,23.83
GPIO26/CAMERA_HREF  (via drill 0.2 layers 1-15)
  Top 0.127: J6.9 18.24,34.59 18.24,33.02 19.5,31.77 19.5,28.63 22.95,25.17 v22.95,25.01
  Route15 0.127: U1.B8 24,22 24,23.96 v22.95,25.01
  other vias: 24.5,21.5
GPIO27/I2C_SCL_CAMERA  (via drill 0.2)
  Top 0.127: U1.B9 24.5,23.7 v24.37,23.83 | J6.5 16.25,33.28 16.76,32.77 16.76,31.75 | R13.1 16.1,31.75 16.76,31.75 | v21.93,24.19 21.93,24.35 16.76,29.53 16.76,31.75
  Bottom 0.127: v24.37,23.83 24,24.2 v21.93,24.2 v21.93,24.19
GPIO28/CAMERA_Y7
  Top 0.127: U1.A9 24,24.16 23.32,24.84 23.32,25.16 19.75,28.73 J6.12
GPIO29/MIC1
  Top 0.127: 13,7.85 R20.1 12.85,11.49 18.25,16.89 18.25,21.52 18.09,21.68 18.09,22.61 17.74,22.95 | U4.7 17.05,23.64 17.74,22.95 | U1.A5 23.56,20 22.52,21.04 22.52,23.07 22.21,23.38 18.17,23.38 17.74,22.95
GPIO33/SWO  (via drill 0.2, 0.2 layers 1-15)
  Top 0.127: J5.6 31.34,29 31.33,29.01 v29.63,29.01
  Route15 0.127: U1.B6 24.37,20.63 24.35,20.63 23.24,21.74 22.79,21.74 21.17,23.35 v21.17,24.14
  Bottom 0.127: v21.17,24.14 22.39,25.36 27.63,25.36 29.63,27.36 v29.63,29.01
  other vias: 24.5,20.5
GPIO36_J3_4  (via drill 0.2, 0.2 layers 1-15)
  Route15 0.127: 27.52,20.48 U1.H6 27.63,20.63 27.65,20.63 27.77,20.75 30.91,20.75 31.88,19.78 v32.89,19.78
  Bottom 0.127: J3.4 29.21,2.54 29.21,6.19 32.89,9.87 v32.89,19.78
  other vias: 27.5,20.5
GPIO37_LED_BLUE  (via drill 0.2, 0.2 layers 1-15)
  Top 0.127: R6.2 17,7.87 v18.09,8.97
  Route15 0.127: U1.H7 31.22,21 v31.95,20.27
  Bottom 0.127: v31.95,20.27 32.01,20.21 32.01,15.08 26.01,9.08 18.2,9.08 v18.09,8.97
  other vias: 27.5,21
GPIO38_J3_3  (via drill 0.2)
  Top 0.127: 28.02,20.48 U1.J6 28.25,20.75 30.39,20.75 v31.43,19.71 | v25.85,9.45 25.85,5.39 26.67,4.57 26.67,2.54 J3.3
  Bottom 0.127: v31.43,19.71 31.76,19.38 31.76,15.51 25.85,9.61 v25.85,9.45
GPIO39_QWIIC_SCK  (via drill 0.2, 0.51)
  Top 0.127: R24.1 35.15,31.34 v35.05,31.24 35.05,30.55 J4.4 37.83,30.5 TP3.P$1 | v34.29,24.38 34.29,24.23 31.79,21.73 28.23,21.73 U1.J8
  Bottom 0.127: v34.29,24.38 34.29,30.48 v35.05,31.24
  other vias: 38.1,30.23
GPIO40_QWIIC_SDA  (via drill 0.51)
  Top 0.127: U1.J9 31.7,22 33.78,24.09 33.78,25.04 | 34.7,25 R23.1 35.11,25.04 33.78,25.04 | 33.78,25.04 33.78,29.21 34.07,29.5 J4.3 36.29,29.5 TP4.P$1
  other vias: 38.1,27.69
GPIO42/I2C_SCLK  (via drill 0.2, 0.2 layers 1-15)
  Top 0.127: R12.1 17.97,12 v18.03,11.94 18.22,11.75 U2.1
  Route15 0.127: v30.76,19.18 30.07,19.87 29.35,19.87 29,20.22 27.97,20.22 27.75,20 U1.H5
  Bottom 0.127: v18.03,11.94 26.9,11.94 30.76,15.8 v30.76,19.17 v30.76,19.18
  other vias: 27.5,20
GPIO43/I2C_SDA  (via drill 0.2)
  Top 0.127: R14.1 17.01,10.16 v18.03,10.16 18.12,10.25 U2.4 | U1.J5 28.44,20 28.57,19.87 30,19.87 30.39,19.48 30.39,19 30.58,18.81 31,18.81 v31.13,18.69
  Bottom 0.127: v18.03,10.16 25.48,10.16 31.13,15.81 v31.13,18.69
GPIO44/LED_GREEN  (via drill 0.2)
  Top 0.127: v32.43,20.36 32.38,20.36 31.74,21 U1.J7 | R8.2 v19.86,8.71
  Bottom 0.127: v32.43,20.36 32.43,20.23 32.27,20.07 32.27,14.97 26.12,8.82 19.98,8.82 v19.86,8.71
GPIO46/LED_RED  (via drill 0.2)
  Top 0.127: R5.2 14.22,8.63 14.22,12.51 18.51,16.79 18.51,21.62 18.45,21.68 v18.45,22.3
  Bottom 0.127: U1.E7 26,22.51 25.79,22.73 18.88,22.73 v18.45,22.3
  other vias: 26,21
GPIO47/LED_YELLOW  (via drill 0.2)
  Top 0.127: U1.H9 27.55,22 27.87,22.32 31.5,22.32 v31.54,22.37 | R7.2 21.02,7.88 21.77,7.88 v21.9,8
  Bottom 0.127: v31.54,22.37 31.54,21.59 32.41,20.73 32.58,20.73 32.8,20.51 32.8,20.21 32.52,19.93 32.52,14.87 26.22,8.57 22.47,8.57 v21.9,8
MIC0_OUT
  Top 0.127: M1.1 8.8,35.9 10,34.7 C24.1
MIC1_OUT
  Top 0.127: M2.1 7.33,4.72 7.6,5 C26.1
N$1
  Top 0.305: L4.2 A1.FEED
N$2
  Top 0.127: U1.G1 27,17.7 27.7,17 28.35,17 Y1.1 29.25,16.1 29.9,16.1 30,16 C7.2
N$3
  Top 0.127: U1.F1 26.5,17.2 27,16.7 27,16 Y1.3 27.9,15.1 C6.2
N$5
  Top 0.127: R6.1 D4.A
N$6
  Top 0.127: R5.1 D3.A
N$7
  Top 0.127: R7.1 D5.A
N$8
  Top 0.127: R8.1 D6.A
N$9
  Top 0.127: U4.5 15.5,21.09 | 15.5,21.09 14.9,21.09 13.63,22.36 U4.3 | R19.2 R18.1 15.5,21.09
N$10
  Top 0.127: C24.2 10.8,31.95 10.8,32.1 11.5,32.8 R16.2
N$11
  Top 0.127: U4.6 17.05,22.36 18,21.41 18,17 11.15,10.15 R20.2 R17.1
N$12  (via drill 0.2 pad 0.25 layers 1-15)
  Top 0.127: U4.2 v12.7,23.64 | v12.57,29.59 R21.2 11.6,31.05 R16.1
  Route15 0.127: v12.7,23.64 12.7,29.46 v12.57,29.59
N$14
  Top 0.127: C26.2 R17.2
N$16
  Top 0.305: L3.2 C18.1 L4.1
RFIOP
  Top 0.305: U1.J1 C17.1 L3.1
SIMBUCK_SWSEL
  Top 0.356: U1.A2 22.57,18.5 22.27,18.8 L1.2
SIMOBUCK_SW
  Top 0.356: U1.A1 23.52,18 22.72,17.2 L1.1
UART-RX/GPIO49  (via drill 0.2, 0.2 pad 0.25 layers 1-15, 0.51)
  Top 0.127: v15.83,23.35 15.83,23.19 15.89,23.13 15.89,22.83 15.67,22.61 13.75,22.61 13.5,22.86 9.12,22.86 7.57,21.3 6.53,21.3 J2.3 5.53,21.27 v4.3,22.5
  Route15 0.127: U1.H8 27.5,21.88 27.51,21.89 27.51,23.34 v27.39,23.46
  Bottom 0.127: v15.83,23.35 15.95,23.46 v27.39,23.46 | v4.3,22.5 4.3,29.99 TP6.P$1
  other vias: 27.5,21.5 3.81,30.48
UART-TX/GPIO48  (via drill 0.2, 0.51)
  Top 0.127: U1.G9 27,22.73 v26.87,22.87 | v15.52,22.98 13.74,22.98 13.61,23.11 9.15,23.11 8.45,23.81 J2.2 5.49,23.81 v4.8,24.5
  Bottom 0.127: v26.87,22.87 26.75,22.98 v15.52,22.98 | v4.8,24.5 4.8,32.03 TP5.P$1
  other vias: 3.81,33.02
V_BATT  (via drill 0.2 pad 0.25)
  Top 0.305: D1.A 9.85,15.15 v12,13
  Bottom 0.127: 12,9.05 BT1.1
  Bottom 0.305: v12,13 12,9.05
VDCDCRF  (via drill 0.2, 0.2 pad 0.25)
  Bottom 0.127: U1.G2 27,18.4 C4.1
  Bottom 0.152: C4.1 27.93,17.48 27.93,16.02 27.1,15.2 R2.2
  other vias: 27,18.5 22.3,15.2
VDD  (via drill 0.2, 0.2 layers 1-15, 0.2 pad 0.25, 0.2 pad 0.25 layers 1-15)
  Top 0.127: U2.2 17.99,11.25 | 17.99,11.25 15.95,11.25 | R12.2 15.2,12 15.95,11.25 | U2.3 18.25,10.75 17.99,11.01 17.99,11.25 | 15.95,11.25 15.15,10.45 R14.2 | U2.10 21.7,11.75 | 21.7,11.75 22.25,11.75 C20.1 | U2.9 21.45,11.25 21.7,11.5 21.7,11.75 | J6.11 19.25,35.75 18.9,36.1 v17,36.1 16.1,36.1 15.75,35.75 J6.4 | v12.15,15.5 D1.C | C21.1 24.13,11.72 24.13,11.43 | U1.J4 v28.77,19.5
  Bottom 0.127: U1.C4 24.88,19.38 C14.1 | 28.2,19.5 28.23,19.5 C15.1 28.43,19.5 v28.77,19.5 | U1.F3 26.48,19 C13.1 | U1.B2 24.25,18.25 C12.1 24.2,18 | 24.2,18 C16.1 | U1.B1 24.2,18
  other vias: 24.5,18.5 25,19.5 26.5,19 8.5,34.5 7.33,35.91 16.8,24.91 16.5,19.5 12.15,18.5 15.15,12 15.15,10 29,32.5 25.55,29.7 22.5,11.5 24,11.85 14.5,30.15 16,30.15 17.5,30.5 9.5,8.5 8.68,4.09 10.5,3.5 24.5,18 36.85,25 35,28.5 36.85,33 32.5,33 0.8,31.5 21.08,14.47 19.05,14.46
  pour Route15 (isolate 0.254): 0,40 0,0 40,0 40,40
VDDBH
  Top 0.127: 24.4,16.28 24.32,16.2
  Top 0.152: 22.45,16.2 R2.1
  Top 0.356: U1.C1 25,16.88 24.4,16.28 L2.2 | 24.32,16.2 C2.1 22.45,16.2
VDDBH_SW
  Top 0.356: U1.D1 25.5,16.87 26,16.37 L2.1
VDDC  (via drill 0.2 pad 0.25)
  Bottom 0.127: C3.1 23.77,19.23 U1.A3
  other vias: 24,19
VDDF  (via drill 0.2 pad 0.25)
  Bottom 0.127: C5.1 25.27,18.27 U1.D2
  other vias: 25.5,18.5
VDDS  (via drill 0.2 pad 0.25)
  Bottom 0.127: C8.1 U1.E1
  other vias: 26,18
X0
  Top 0.127: C10.2 21.05,22.8 Y2.P$1 21.3,21.03 21.51,20.82 22.25,20.82 22.42,20.65 22.42,19.8 22.71,19.5 U1.A4
XI  (via drill 0.2 layers 1-15)
  Top 0.127: C9.2 21.05,19.8 Y2.P$2
  Route15 0.127: U1.B4 21.85,19.5 Y2.P$2
  other vias: 24.5,19.5 21.3,20.05

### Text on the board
Bottom: v01
tDocu: This is a 4-layer board! | Jim Lindblom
